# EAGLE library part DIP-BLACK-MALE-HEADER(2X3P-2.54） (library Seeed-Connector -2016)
320020077
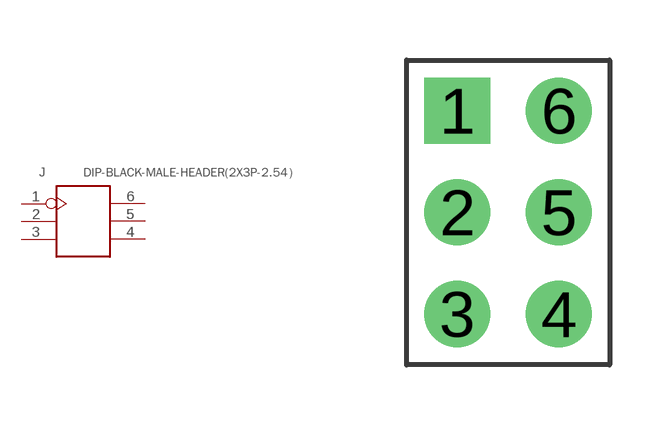
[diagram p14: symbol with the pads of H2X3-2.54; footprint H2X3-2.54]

Designator prefix J

## DIP-BLACK-MALE-HEADER(2X3P-2.54）-2.54 (MPN: P125-12A1BS116A1; VALUE: 2x3p-2.54)  [H2X3-2.54]
1  1
2  2
3  3
4  4
5  5
6  6

## Footprint H2X3-2.54 (pad centres in mm)
drill 0.889 pad 1.651 square: 1 -1.27,2.54
drill 0.889 pad 1.651: 2 -1.27,0; 3 -1.27,-2.54; 4 1.27,-2.54; 5 1.27,0; 6 1.27,2.54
